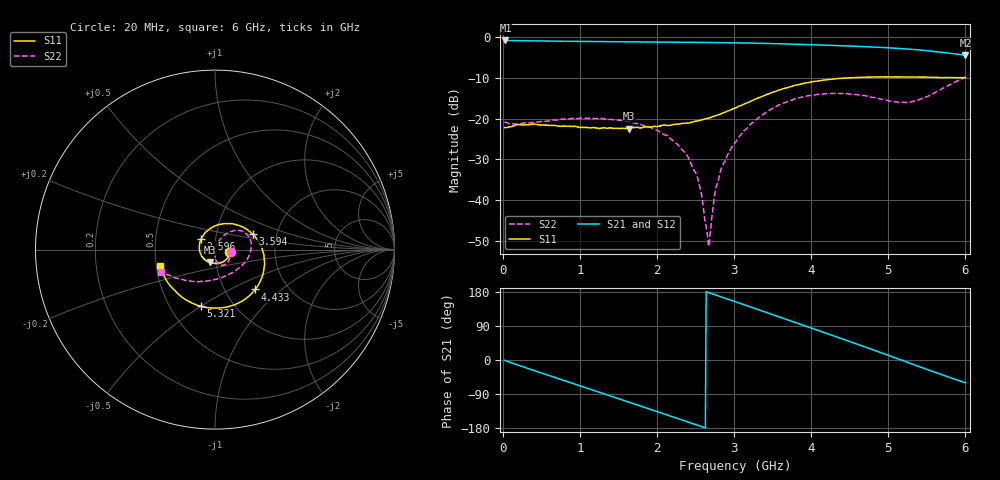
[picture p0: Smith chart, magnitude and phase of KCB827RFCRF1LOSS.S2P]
!Agilent Technologies,E5071B,JP1KK00126,A.08.11
!Date: Tue May 06 07:33:46 2014
!Data & Calibration Information:
!Freq	S11:SOLT2(ON)	S21:SOLT2(ON)	S12:SOLT2(ON)	S22:SOLT2(ON)
# Hz S dB R 50
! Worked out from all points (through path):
!   600 points, 20 MHz to 6 GHz, reference 50 ohm
!   highest |S21| = -0.78 dB at 29.98 MHz (marker M1); lowest = -4.4 dB at 6 GHz (marker M2)
!   group delay of S21, straight-line fit = 194 ps
!   lowest |S11| = -22.5 dB at 1.637 GHz (marker M3), VSWR 1.16, Z = 46.6 - j6.45 ohm
!   |S11| at or under -10 dB: start of sweep to 4.438 GHz
!   |S22| runs from -51.3 to -9.8 dB; largest |S21 - S12| = 0.0045
!   S11 on the Smith chart (normalised r, x): 20 MHz: 1.16, -0.04; 2.596 GHz: 0.85, +0.10; 3.594 GHz: 1.50, +0.27; 4.433 GHz: 1.38, -0.68; 5.321 GHz: 0.71, -0.50; 6 GHz: 0.52, -0.10
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2e7  -22.17 -11.2  -0.78 -0.5  -0.77 -0.6  -20.75 -8.7
2.998331e7  -22.19 -8.6  -0.78 -1.6  -0.77 -1.6  -20.86 -6.2
4.892154e8  -21.56 -34.7  -0.90 -33.7  -0.91 -33.8  -20.71 -24.9
1.018331e9  -22.11 -70.2  -1.01 -69.6  -1.01 -69.6  -19.84 -48.2
1.637295e9  -22.49 -113.7  -1.12 -111.6  -1.11 -111.7  -20.77 -71.5
2.016661e9  -21.87 -146.4  -1.17 -137.5  -1.17 -137.5  -23.04 -81.5
2.386043e9  -21.06 171.3  -1.23 -162.8  -1.23 -162.9  -28.95 -88.2
2.52581e9  -20.52 152.0  -1.25 -172.4  -1.25 -172.6  -34.60 -88.3
2.595693e9  -20.14 141.8  -1.27 -177.1  -1.26 -177.4  -41.28 -83.8
2.645609e9  -19.94 135.3  -1.27 179.4  -1.28 179.2  -47.88 -63.1
2.675559e9  -19.82 131.2  -1.27 177.1  -1.28 177.1  -51.32 25.3
2.745442e9  -19.36 121.8  -1.28 172.3  -1.29 172.3  -38.75 62.0
2.795359e9  -19.06 114.5  -1.29 168.9  -1.31 168.8  -35.01 68.7
3.014992e9  -17.36 86.2  -1.35 153.6  -1.35 153.5  -25.84 65.2
3.234624e9  -15.53 59.8  -1.44 138.3  -1.43 138.1  -21.04 58.6
3.594023e9  -12.90 22.4  -1.60 112.8  -1.59 112.8  -16.56 45.3
4.013322e9  -10.93 -13.9  -1.83 83.2  -1.84 83.2  -14.20 27.4
4.432621e9  -10.01 -44.7  -2.10 53.4  -2.11 53.4  -13.82 5.2
5.011653e9  -9.73 -82.4  -2.59 11.3  -2.59 11.3  -15.66 -42.0
5.321135e9  -9.76 -104.0  -2.98 -11.6  -2.98 -11.7  -15.74 -84.0
5.650584e9  -9.86 -130.8  -3.61 -35.8  -3.59 -35.8  -13.12 -127.1
6e9  -9.89 -163.9  -4.39 -60.3  -4.39 -60.3  -9.78 -157.7
